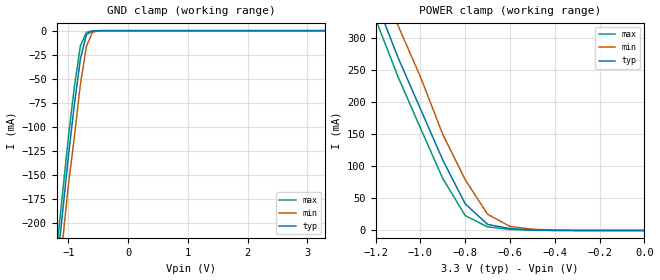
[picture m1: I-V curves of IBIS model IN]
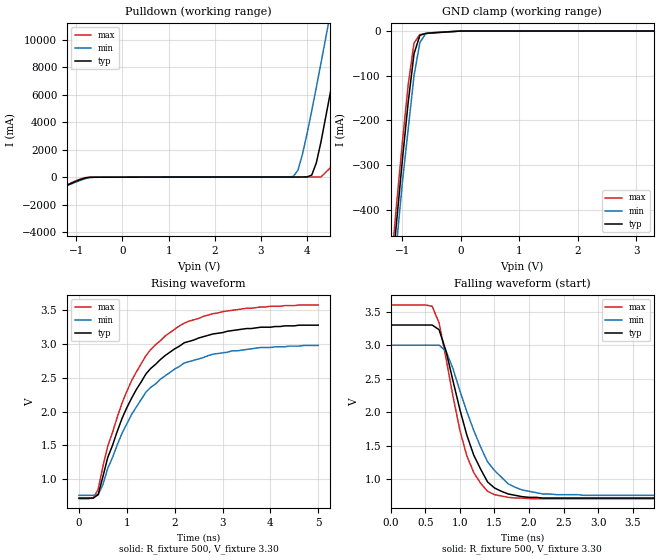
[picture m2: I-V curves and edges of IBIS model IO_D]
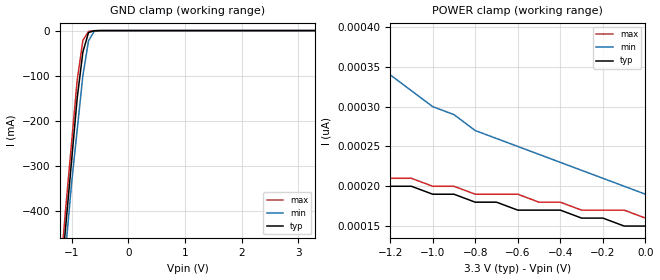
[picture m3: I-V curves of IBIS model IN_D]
| Integrated Devices Technolgy, Inc
[Ibis Ver]   3.2
[File Name]   9zx21901d.ibs
[File Rev]   1.1
[Date]   Tuesday, March 16, 2010
[Source]   Integrated Devices Technolgy, Inc.
[Notes]   Rev 1.0 created by wm
|   March 16, 2010
|   Updated by LP April 5, 2010
|   Added Vmeas, Cref, Rref, Vref parameters. Correct Diff_Pin
[Disclaimer] Integrated Device Technology, Inc. ("IDT") hereby grants the
   user of this IBIS model a non-exclusive, nontransferable
   license to use this IBIS model under the following terms. The
   user is granted this license only to use the IBIS model and is
   not granted rights to sell, copy (except as needed to run the
   IBIS model), rent, lease or sub-license the IBIS model in
   whole or in part, or in modified form to anyone. The User may
   modify the IBIS model to suit its specific applications, but
   rights to derivative works and such modifications shall belong
   to IDT. This IBIS model is provided on an AS IS" basis and IDT
   makes absolutely no warranty with respect to the information
   contained herein. IDT DISCLAIMS AND CUSTOMER WAIVES ALL
   WARRANTIES, EXPRESS AND IMPLIED, INCLUDING WARRANTIES OF
   MERCHANTABILITY AND FITNESS FOR A PARTICULAR PURPOSE. THE
   ENTIRE RISK AS TO QUALITY AND PERFORMANCE IS WITH THE USER
   ACCORDINGLY, IN NO EVENT SHALL IDT BE LIABLE FOR ANY DIRECT OR
   INDIRECT DAMAGES, WHETHER IN CONTRACT OR TORT, INCLUDING ANY
   LOST PROFITS OR OTHER INCIDENTAL, CONSEQUENTIAL, EXEMPLARY, OR
   PUNITIVE DAMAGES ARISING OUT OF THE USE OR APPLICATION OF THE
   IBIS model. Further, IDT reserves the right to make changes
   without notice to any product herein to improve reliability,
   function, or design. IDT does not convey any license under
   patent rights or any other intellectual property rights,
   including those of third parties. IDT is not obligated to
   provide maintenance or support for the licensed IBIS model.
[Disclaimer]   (C) Copyright Integrated Device Technology, Inc. 2010 All
   rights reserved
|   COMPONENT: ICS9ZX21901D
[Component]   ICS9ZX21901D
[Manufacturer]   Integrated Device Technology, Inc.
[Package]
| variable   typ   min   max
R_pkg   81.10m   62.20m   100.00m
L_pkg   6.70nH   4.90nH   8.50nH
C_pkg   0.53pF   0.21pF   0.85pF
[Pin]   signal_name   model_name   R_pin   L_pin   C_pin
1   VDDA   POWER
2   GNDA   GND
3   IREF   NC
4   100M_133M#   IN
5   HIBW_BYPM_LOBW#   IN
6   CK_POWERGD/PD#   IN
7   GND   GND
8   VDD   POWER
9   DIF_IN   DIFF_IN
10   DIF_IN#   DIFF_IN
11   SMB_A0_tri   IN
12   SMBDAT   IO_D
13   SMBCLK   IN_D
14   SMB_A1_tri   IN
15   NC   NC
16   NC   NC
17   DFB_OUT#   OUT
18   DFB_OUT   OUT
19   DIF_0   OUT
20   DIF_0#   OUT
21   VDD   POWER
22   DIF_1   OUT
23   DIF_1#   OUT
24   DIF_2   OUT
25   DIF_2#   OUT
26   GND   GND
27   DIF_3   OUT
28   DIF_3#   OUT
29   DIF_4   OUT
30   DIF_4#   OUT
31   VDD   POWER
32   DIF_5   OUT
33   DIF_5#   OUT
34   OE5#   IN
35   DIF_6   OUT
36   DIF_6#   OUT
37   OE6#   IN
38   DIF_7   OUT
39   DIF_7#   OUT
40   OE7#   IN
41   DIF_8   OUT
42   DIF_8#   OUT
43   OE8#   IN
44   GND   GND
45   VDD   POWER
46   DIF_9   OUT
47   DIF_9#   OUT
48   OE9#   IN
49   DIF_10   OUT
50   DIF_10#   OUT
51   OE10#   IN
52   DIF_11   OUT
53   DIF_11#   OUT
54   OE_11#   IN
55   DIF_12   OUT
56   DIF_12#   OUT
57   OE12#   IN
58   VDD   POWER
59   DIF_13   OUT
60   DIF_13#   OUT
61   DIF_14   OUT
62   DIF_14#   OUT
63   GND   GND
64   DIF_15   OUT
65   DIF_15#   OUT
66   DIF_16   OUT
67   DIF_16#   OUT
68   VDD   POWER
69   DIF_17   OUT
70   DIF_17#   OUT
71   DIF_18   OUT
72   DIF_18#   OUT
[Diff Pin]   inv_pin   vdiff   tdelay_typ
9   10   NA   NA
18   17   NA   NA
19   20   NA   NA
22   23   NA   NA
24   25   NA   NA
27   28   NA   NA
29   30   NA   NA
32   33   NA   NA
35   36   NA   NA
38   39   NA   NA
41   42   NA   NA
46   47   NA   NA
49   50   NA   NA
52   53   NA   NA
55   56   NA   NA
59   60   NA   NA
61   62   NA   NA
64   65   NA   NA
66   67   NA   NA
69   70   NA   NA
71   72   NA   NA
[Model Selector] OUT
OUT_slow_475   100ohm differential output trace. 475ohm on IREF pin.
OUT_slow_432   85ohm differential output trace. 432ohm on IREF pin.
OUT_slow_412   85ohm differential output trace. 412ohm on IREF pin.
| Models and submodels in the file (7): IN (Input), DIFF_IN (Input), IO_D (I/O_open_drain), IN_D (Input), OUT_slow_475 (Open_source), OUT_slow_412 (Open_source), OUT_slow_432 (Open_source)
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|   Model IN
[Model]   IN
Model_type   Input
Polarity   Inverting
Enable   Active-High
Vinl =   1.00V
Vinh =   2.00V
C_comp   3.40pF   2.85pF   3.95pF
[Temperature Range]   27.00   70.00   0.000
[Voltage Range]   3.30V   3.00V   3.60V
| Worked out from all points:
|   GND clamp passes 1 mA (typ) near -0.62 V on its own axis
|   POWER clamp passes 1 mA (typ) near -0.51 V on its own axis
[GND_clamp]
| voltage   I(typ)   I(min)   I(max)
-3.3V     -1.54A     -1.54A     -1.54A
-1.2V     -250mA     -270mA     -230mA
-1.1V     -190mA     -220mA     -170mA
-1V       -130mA     -160mA     -110mA
-900mV    -75.97mA   -110mA     -57.72mA
-800mV    -29.3mA    -55.39mA   -15.7mA
-700mV    -4.2mA     -16.67mA   -1.77mA
-600mV    -420uA     -1.81mA    -210uA
-500mV    -36.28uA   -150uA     -14.74uA
3.3V      150pA      92.22uA    -1.21nA
[POWER_clamp]
| voltage   I(typ)   I(min)   I(max)
-3.3V     2.31A      2.35A      2.29A
-1.2V     360mA      410mA      330mA
-1.1V     270mA      320mA      240mA
-1V       190mA      240mA      160mA
-900mV    110mA      150mA      81.19mA
-800mV    41.59mA    79.25mA    23.27mA
-700mV    9.51mA     25.32mA    5.62mA
-600mV    2.91mA     6.31mA     1.67mA
-500mV    750uA      1.96mA     350uA
-300mV    20.87uA    92.22uA    6.56uA
0V        150pA      200pA      160pA
|   Model IO_D
[Model]   IO_D
Model_type   I/O_open_drain
Polarity   Non-Inverting
Enable   Active-High
Vinl =   .300V
Vinh =   2.00V
Vmeas =   0.350V
Cref =   2.00pF
Rref =   0.000
Vref =   0.350V
C_comp   3.40pF   2.85pF   3.95pF
[Temperature Range]   27.00   70.00   0.000
[Voltage Range]   3.30V   3.00V   3.60V
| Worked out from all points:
|   slope of the pulldown table from 0 to 0.495 V, typ, clamps not added: 131 ohm
|   GND clamp passes 1 mA (typ) near -0.12 V on its own axis
|   rising waveform, R_fixture 500, V_fixture 3.30: 20-80 % time 1.13ns typ, 1.18ns min, 1.1ns max; typ from 0.72 V to 3.28 V
|   falling waveform, R_fixture 500, V_fixture 3.30: 20-80 % time 430ps typ, 510ps min, 367ps max; typ from 3.3 V to 0.72 V
[Pulldown]
| voltage   I(typ)   I(min)   I(max)
-3.3V     -3.78A     -3.65A     -3.87A
-800mV    -50.99mA   -100mA     -26.91mA
3.7V      9.44mA     53.55mA    11.23mA
3.8V      10.07mA    490mA      11.25mA
3.9V      12.32mA    1.67A      11.27mA
4.1V      150mA      4.83A      11.65mA
4.3V      2.56A      8.29A      17.33mA
4.5V      6.09A      11.85A     670mA
4.7V      9.81A      15.47A     3.91A
4.9V      13.62A     19.11A     7.69A
5.1V      17.46A     22.78A     11.6A
6.6V      46.76A     50.55A     41.81A
[GND_clamp]
| voltage   I(typ)   I(min)   I(max)
-3.3V     -3.78A     -3.65A     -3.87A
-1.2V     -570mA     -610mA     -540mA
-1.1V     -430mA     -480mA     -390mA
-1V       -290mA     -340mA     -250mA
-900mV    -160mA     -220mA     -120mA
-800mV    -50.99mA   -100mA     -26.91mA
-700mV    -9.68mA    -25.77mA   -7.84mA
-600mV    -5.33mA    -5.93mA    -5.63mA
0V        0A         0A         0A
3.3V      150pA      220pA      150pA
[Ramp]
| variable   typ   min   max
dV/dt_r   1.54/1.11n   1.33/1.16n   1.72/1.07n
dV/dt_f   1.55/0.42n   1.34/0.53n   1.73/0.36n
R_load = 500
[Rising Waveform]
R_fixture = 500
V_fixture = 3.30
V_fixture_min = 3.00
V_fixture_max = 3.60
| time   V(typ)   V(min)   V(max)
0s        720mV      760mV      710mV
300ps     720mV      760mV      720mV
400ps     770mV      770mV      850mV
600ps     1.32V      1.16V      1.49V
1ns       2.06V      1.82V      2.3V
1.4ns     2.56V      2.29V      2.83V
1.8ns     2.83V      2.53V      3.12V
2.2ns     3.02V      2.72V      3.31V
3ns       3.17V      2.87V      3.48V
5ns       3.28V      2.98V      3.58V
[Falling Waveform]
R_fixture = 500
V_fixture = 3.30
V_fixture_min = 3.00
V_fixture_max = 3.60
| time   V(typ)   V(min)   V(max)
0s        3.3V       3V         3.6V
600ps     3.3V       3V         3.58V
700ps     3.23V      3V         3.33V
800ps     2.91V      2.91V      2.8V
1ns       2.04V      2.32V      1.73V
1.1ns     1.66V      2.01V      1.35V
1.4ns     960mV      1.26V      820mV
1.7ns     780mV      930mV      730mV
2.2ns     720mV      780mV      710mV
5ns       720mV      760mV      710mV
|   Model IN_D
[Model]   IN_D
Model_type   Input
Polarity   Inverting
Enable   Active-High
Vinl =   1.00V
Vinh =   2.00V
C_comp   3.40pF   2.85pF   3.95pF
[Temperature Range]   27.00   70.00   0.000
[Voltage Range]   3.30V   3.00V   3.60V
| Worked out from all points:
|   GND clamp passes 1 mA (typ) near -0.62 V on its own axis
[GND_clamp]
| voltage   I(typ)   I(min)   I(max)
-3.3V     -3.78A     -3.65A     -3.87A
-1.2V     -570mA     -610mA     -540mA
-1.1V     -430mA     -480mA     -390mA
-1V       -290mA     -340mA     -250mA
-900mV    -150mA     -220mA     -110mA
-800mV    -47.77mA   -100mA     -21.77mA
-700mV    -4.42mA    -22.5mA    -1.71mA
-600mV    -390uA     -1.83mA    -190uA
-500mV    -33.14uA   -140uA     -13.41uA
3.3V      150pA      220pA      150pA
[POWER_clamp]
| voltage   I(typ)   I(min)   I(max)
-3.3V     350pA      1.67nA     300pA
-2.6V     280pA      890pA      270pA
-2.5V     280pA      820pA      260pA
-2.3V     260pA      700pA      260pA
-2.2V     250pA      640pA      250pA
-1.5V     220pA      400pA      220pA
-1.4V     210pA      380pA      220pA
-1V       190pA      300pA      200pA
-800mV    180pA      270pA      190pA
-600mV    170pA      250pA      190pA
-400mV    170pA      230pA      180pA
0V        150pA      190pA      160pA
